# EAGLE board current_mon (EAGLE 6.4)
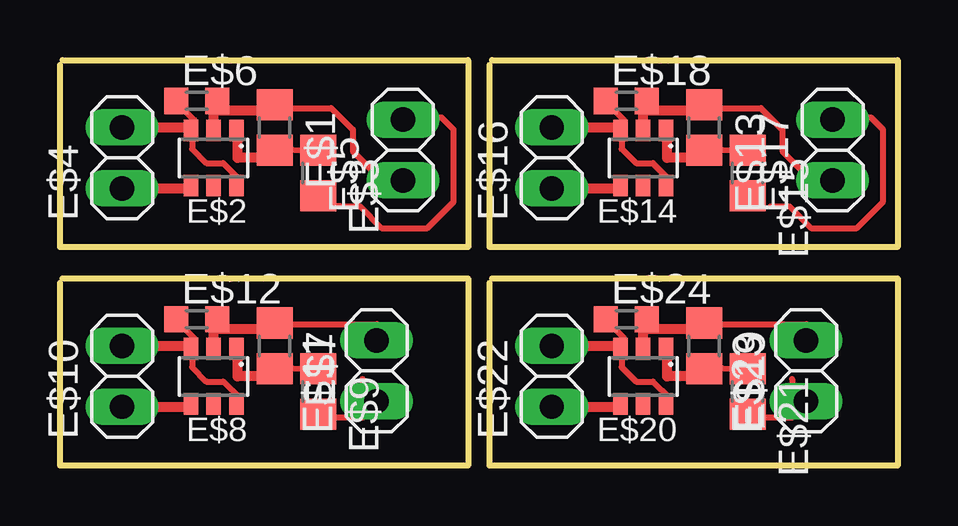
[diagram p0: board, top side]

Size 34.9 x 16.9 mm. Coordinates in mm from the lower left corner, seen from the top.
Outline: 0.1,16.9 17,16.9 17,9.1 0,9.1 0,16.7
Outline: 0.1,7.8 17,7.8 17,0 0,0 0,7.6
Outline: 18,16.9 34.9,16.9 34.9,9.1 17.9,9.1 17.9,16.7
Outline: 18,7.8 34.9,7.8 34.9,0 17.9,0 17.9,7.6
Copper layers (1*16): Top 0.035mm / dielectric 1.5mm / Bottom 0.035mm
Design rules "default": minimum track width 10mil, minimum drill 24mil, track to track 8mil, track to pad 8mil, pad to pad 8mil, via to via 8mil, smd to smd 8mil, copper to edge 40mil, drill to drill 8mil, minimum pad ring 10mil, minimum via ring 8mil, stop-mask expansion 4mil, vias tented up to drill 0mil, thermal gap 10mil

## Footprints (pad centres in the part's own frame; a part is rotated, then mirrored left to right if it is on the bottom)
R0805 = smd 1.3 x 1.5: 1 -0.95,0; 2 0.95,0
SOT23-6 = smd 0.6 x 0.9: 1 -0.95,-1.15; 2 0,-1.15; 3 0.95,-1.15; 4 0.95,1.15; 5 0,1.15; 6 -0.95,1.15
1X02 = drill 1.016 long: 1 -1.27,0; 2 1.27,0
R0603 = smd 1 x 1.1: 1 -0.85,0; 2 0.85,0

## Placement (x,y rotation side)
E$1  [R0805]  8.94,14.09 270 top
E$2  [SOT23-6]  6.4,12.82 180 top
E$3  [R0805]  10.75,12.19 270 top
E$4  [1X02]  2.59,12.82 90 top
E$5  [1X02]  14.29,13.15 90 top
E$6  [R0603]  5.7,15.2 0 top
E$7  [R0805]  8.94,4.99 270 top
E$8  [SOT23-6]  6.4,3.72 180 top
E$9  [R0805]  10.75,3.09 270 top
E$10  [1X02]  2.59,3.72 90 top
E$11  [1X02]  13.19,3.95 90 top
E$12  [R0603]  5.7,6.1 0 top
E$13  [R0805]  26.84,14.09 270 top
E$14  [SOT23-6]  24.3,12.82 180 top
E$15  [R0805]  28.65,12.19 270 top
E$16  [1X02]  20.49,12.82 90 top
E$17  [1X02]  32.19,13.15 90 top
E$18  [R0603]  23.6,15.2 0 top
E$19  [R0805]  26.84,4.99 270 top
E$20  [SOT23-6]  24.3,3.72 180 top
E$21  [R0805]  28.65,3.09 270 top
E$22  [1X02]  20.49,3.72 90 top
E$23  [1X02]  31.09,3.95 90 top
E$24  [R0603]  23.6,6.1 0 top

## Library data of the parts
E$1 E$3 E$7 E$9 E$13 E$15 E$19 E$21 = rcl
E$2 E$8 E$14 E$20 = linear
E$4 E$5 E$10 E$11 E$16 E$17 E$22 E$23 = pinhead
E$6 E$12 E$18 E$24 = eagle-ltspice

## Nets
S$1: E$4.1
S$2: E$4.2
S$11: E$10.1
S$14: E$10.2
S$25: E$16.1
S$26: E$16.2
S$35: E$22.1
S$36: E$22.2

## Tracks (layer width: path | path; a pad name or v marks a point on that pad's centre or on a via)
S$1
  Top 0.406: E$4.1 5.13,11.55
S$2
  Top 0.406: E$4.2 5.13,14.09
S$3
  Top 0.406: 8.94,12.82 7.4,12.82 7.4,14
S$4
  Top 0.406: 6.3,14.2 6.4,14.2 6.4,14.8 8.9,14.8 8.9,14.7
S$5
  Top 0.406: 9,14.8 9,14.9
S$6
  Top 0.254: 14.3,14.4 14.4,14.5 15.9,14.5 16.4,14 16.4,11 15.3,9.9 13.4,9.9 12.5,10.8 11.8,10.8 11.7,10.8 11,10.8 10.9,10.9
S$7
  Top 0.254: 9.1,13.2 10.7,13.1
S$8
  Top 0.254: 5.1,14.9 5.6,14.4 5.6,14.1 5.5,14
S$9
  Top 0.254: 9.5,12.6 9.4,12.7
S$10
  Top 0.254: 9.2,14.9 11.3,14.9 12.2,14 12.2,13.1 13.2,12.1 14.3,12.1 14.4,12
S$11
  Top 0.406: E$10.1 5.13,2.45
S$12
  Top 0.254: 7.5,11.6 7.4,11.5
S$13
  Top 0.254: 7.5,11.9 6.8,12.6 6.1,12.6 5.5,13.2 5.5,13.9
S$14
  Top 0.406: E$10.2 5.13,4.99
S$15
  Top 0.406: 8.94,3.72 7.4,3.72 7.4,4.9
S$16
  Top 0.406: 6.3,5.1 6.4,5.1 6.4,5.7 8.9,5.7 8.9,5.6
S$17
  Top 0.406: 9,5.7 9,5.8
S$18
  Top 0.254: 9.5,3.5 9.4,3.6
S$19
  Top 0.254: 5.1,5.8 5.6,5.3 5.6,5 5.5,4.9
S$20
  Top 0.254: 7.5,2.8 6.8,3.5 6.1,3.5 5.5,4.1 5.5,4.8
S$21
  Top 0.254: 7.5,2.5 7.4,2.4
S$22
  Top 0.254: 9.1,4.1 10.7,4
S$23
  Top 0.254: 12.6,3.6 12.6,2 10.8,2
S$24
  Top 0.254: 8.9,5.9 13.2,5.9 13.2,5.1
S$25
  Top 0.406: E$16.1 23.03,11.55
S$26
  Top 0.406: E$16.2 23.03,14.09
S$27
  Top 0.406: 26.84,12.82 25.3,12.82 25.3,14
S$28
  Top 0.406: 24.2,14.2 24.3,14.2 24.3,14.8 26.8,14.8 26.8,14.7
S$29
  Top 0.406: 26.9,14.8 26.9,14.9
S$30
  Top 0.254: 27.4,12.6 27.3,12.7
S$31
  Top 0.254: 23,14.9 23.5,14.4 23.5,14.1 23.4,14
S$32
  Top 0.254: 25.4,11.9 24.7,12.6 24,12.6 23.4,13.2 23.4,13.9
S$33
  Top 0.254: 25.4,11.6 25.3,11.5
S$34
  Top 0.254: 27,13.2 28.6,13.1
S$35
  Top 0.406: E$22.1 23.03,2.45
S$36
  Top 0.406: E$22.2 23.03,4.99
S$37
  Top 0.406: 26.84,3.72 25.3,3.72 25.3,4.9
S$38
  Top 0.406: 24.2,5.1 24.3,5.1 24.3,5.7 26.8,5.7 26.8,5.6
S$39
  Top 0.406: 26.9,5.7 26.9,5.8
S$40
  Top 0.254: 27.4,3.5 27.3,3.6
S$41
  Top 0.254: 23,5.8 23.5,5.3 23.5,5 23.4,4.9
S$42
  Top 0.254: 25.4,2.8 24.7,3.5 24,3.5 23.4,4.1 23.4,4.8
S$43
  Top 0.254: 25.4,2.5 25.3,2.4
S$44
  Top 0.254: 27,4.1 28.6,4
S$45
  Top 0.254: 30.5,3.6 30.5,2 28.7,2
S$46
  Top 0.254: 26.8,5.9 31.1,5.9 31.1,5.1
S$47
  Top 0.254: 29.6,10.8 30.4,10.8 31.3,9.9 33.2,9.9 34.3,11 34.3,14 33.8,14.5 32.3,14.5 32.2,14.4
S$48
  Top 0.254: 27.1,14.9 29.2,14.9 30.1,14 30.1,13.1 31.1,12.1 32.2,12.1 32.3,12

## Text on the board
tDocu: VCC C 1nF RL GND / GND SO8 R_SCHUTZ V_AD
